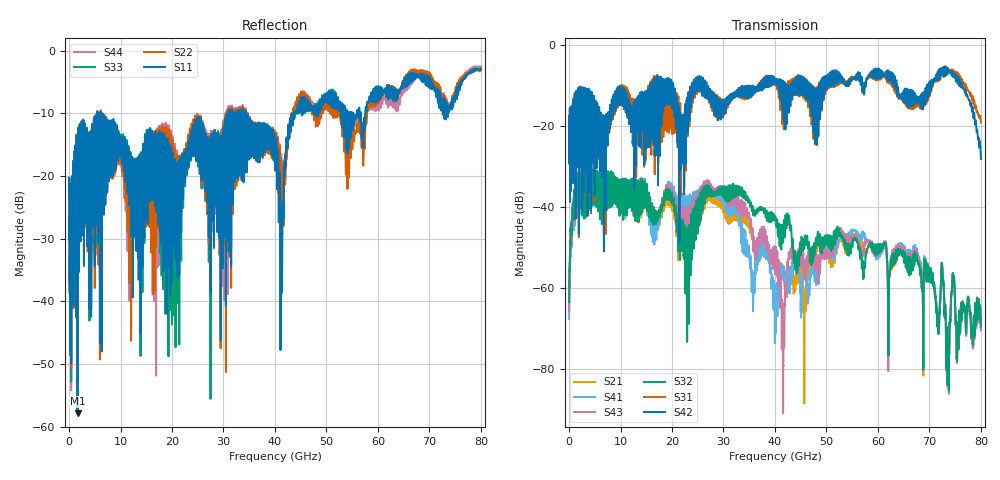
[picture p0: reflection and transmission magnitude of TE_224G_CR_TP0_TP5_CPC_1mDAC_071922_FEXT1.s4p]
!! Reference: tracy_3df_01a_2207
!! CHANNEL DESCRIPTION: TP0_TP5 CR Channel using 1meter DAC, CABLED CPC Host
!! MODEL DESCRIPTION: s4p, FEXT1
!! CONNECTOR DESCRIPTION: OSFP 200G OTB, CPC Socket
!! CABLE DESCRIPTION: 1meter 26AWG Cable
!! MODEL STATUS: Developmental
!! PORT DEFINITIONS:
!! Port  1  ----->  Side A  Side B  <-----  Port  2
!! Port  3  ----->  Side A  Side B  <-----  Port  4
# GHz S MA R 50
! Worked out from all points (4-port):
!   8000 points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, 10 MHz to 80 GHz, reference 50 ohm
!   strongest paths, dB at 10 MHz, 20.01 GHz, 40.01 GHz, 60.01 GHz, 80 GHz:
!     S42: -24.6, -14.4, -9.7, -7.8, -28.3
!     S31: -24.6, -20.2, -10.1, -8.2, -19.3
!     S32: -63.6, -37.7, -42.7, -51.4, -69.7
!     S43: -65.9, -36.5, -56.7, -51.7, -70.5
!     S41: -67.8, -35.5, -62.4, -52.6, -70.5
!     S21: -65.9, -39.1, -54.2, -52.2, -69.7
!   lowest |S11| = -57.8 dB at 1.64 GHz (marker M1), VSWR 1.00, Z = 49.9 - j0.00388 ohm
!   |S11| at or under -10 dB: start of sweep to 5.488 GHz; 6.171 GHz to 30.97 GHz (24.8 GHz wide, 134 % of centre); 34.4 GHz to 43.55 GHz (9.158 GHz wide, 23.5 % of centre)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
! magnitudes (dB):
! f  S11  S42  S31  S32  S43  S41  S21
! 10 MHz  -23.3  -24.6  -24.6  -63.6  -65.9  -67.8  -65.9
! 1.64 GHz  -57.8  -19.6  -19.6  -34.5  -35.9  -37.7  -35.9
! 31.82 GHz  -22.6  -13.1  -13.0  -34.3  -35.4  -37.7  -38.5
! 41.57 GHz  -23.9  -9.2  -11.4  -48.5  -87.1  -56.7  -57.1
! 67.23 GHz  -4.3  -12.4  -13.4  -51.2  -50.3  -49.5  -50.4
! 73.24 GHz  -10.9  -5.4  -5.5  -73.6  -73.8  -73.9  -73.7
! 80 GHz  -2.9  -28.3  -19.3  -69.7  -70.5  -70.5  -69.7
